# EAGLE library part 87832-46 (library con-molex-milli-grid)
HEADER
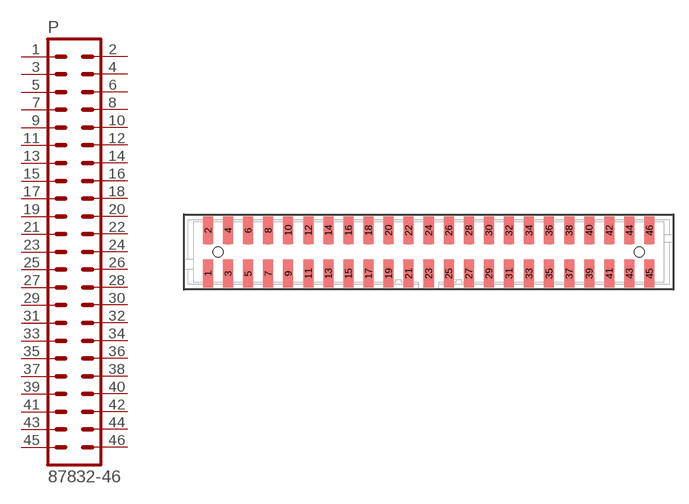
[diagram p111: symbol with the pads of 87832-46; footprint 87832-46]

Designator prefix P

## 87832-46  [87832-46]
1  1  pas
2  2  pas
3  3  pas
4  4  pas
5  5  pas
6  6  pas
7  7  pas
8  8  pas
9  9  pas
10  10  pas
11  11  pas
12  12  pas
13  13  pas
14  14  pas
15  15  pas
16  16  pas
17  17  pas
18  18  pas
19  19  pas
20  20  pas
21  21  pas
22  22  pas
23  23  pas
24  24  pas
25  25  pas
26  26  pas
27  27  pas
28  28  pas
29  29  pas
30  30  pas
31  31  pas
32  32  pas
33  33  pas
34  34  pas
35  35  pas
36  36  pas
37  37  pas
38  38  pas
39  39  pas
40  40  pas
41  41  pas
42  42  pas
43  43  pas
44  44  pas
45  45  pas
46  46  pas

## Footprint 87832-46 (pad centres in mm)
HEADER SMD Dual Row, Shrouded, Vertical
smd 1 x 2.75: 1 -22,-2.15; 2 -22,2.15; 3 -20,-2.15; 4 -20,2.15; 5 -18,-2.15; 6 -18,2.15; 7 -16,-2.15; 8 -16,2.15; 9 -14,-2.15; 10 -14,2.15; 11 -12,-2.15; 12 -12,2.15; 13 -10,-2.15; 14 -10,2.15; 15 -8,-2.15; 16 -8,2.15; 17 -6,-2.15; 18 -6,2.15; 19 -4,-2.15; 20 -4,2.15; 21 -2,-2.15; 22 -2,2.15; 23 0,-2.15; 24 0,2.15; 25 2,-2.15; 26 2,2.15; 27 4,-2.15; 28 4,2.15; 29 6,-2.15; 30 6,2.15; 31 8,-2.15; 32 8,2.15; 33 10,-2.15; 34 10,2.15; 35 12,-2.15; 36 12,2.15; 37 14,-2.15; 38 14,2.15; 39 16,-2.15; 40 16,2.15; 41 18,-2.15; 42 18,2.15; 43 20,-2.15; 44 20,2.15; 45 22,-2.15; 46 22,2.15
hole 1 at -21,0
hole 1 at 21,0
